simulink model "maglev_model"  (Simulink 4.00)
settings: Solver=ode45  StartTime=0.0  StopTime=10.0  RelTol=1e-3
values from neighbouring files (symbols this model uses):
  C = C * 1e-5    [maglev_init.m]
  g = 9.80665    [maglev_init.m]
  L1 = L1/10    [maglev_init.m]
  m = m/100    [maglev_init.m]
  R = input('Inserire le prime due cifre (esclusi zeri) del proprio numero di matricola:\n\n')    [maglev_init.m]
  x1_0 = 0.1    [maglev_init.m]
  x2_0 = 0    [maglev_init.m]
  x3_0 = 0.2    [maglev_init.m]

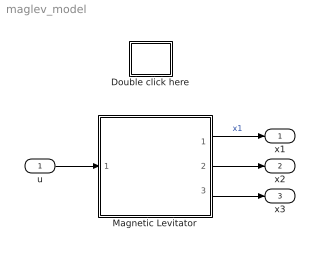
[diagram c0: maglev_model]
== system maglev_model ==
  u : Inport  Port=1  LatchInput=off
  Double click here : Subsystem
  Magnetic Levitator : Subsystem  mask{m=m, R=R, L1=L1, C=C, g=g}
      mask prompts: m "ball's mass (m)"; R "Electromagnet's resistance (R)"; L1 "Electromagnet's inductance (L1)"; C "Magnetic force constant (C)"; g "Gravitational acceleration (g)"
  x1 : Outport  Port=1
  x2 : Outport  Port=2
  x3 : Outport  Port=3
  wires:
  u/1 -> Magnetic Levitator/1(u)
  Magnetic Levitator/1(x1) -> x1/1  "x1"
  Magnetic Levitator/2(x2) -> x2/1
  Magnetic Levitator/3(x3) -> x3/1

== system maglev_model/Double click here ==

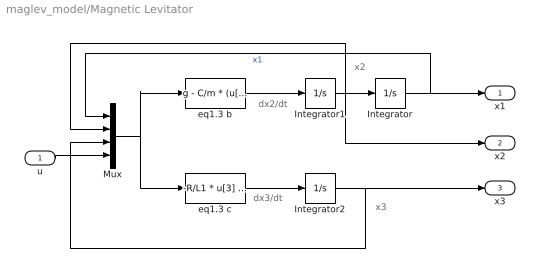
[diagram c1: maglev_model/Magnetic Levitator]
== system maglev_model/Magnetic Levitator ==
  note: x2
  note: x3
  note: dx2/dt
  note: dx3/dt
  u : Inport  Port=1  LatchInput=off
  Integrator : Integrator  ExternalReset=none  InitialConditionSource=internal  InitialCondition=x1_0  LimitOutput=off  UpperSaturationLimit=inf  LowerSaturationLimit=-inf  ShowSaturationPort=off  ShowStatePort=off  AbsoluteTolerance=auto
  Integrator1 : Integrator  ExternalReset=none  InitialConditionSource=internal  InitialCondition=x2_0  LimitOutput=off  UpperSaturationLimit=inf  LowerSaturationLimit=-inf  ShowSaturationPort=off  ShowStatePort=off  AbsoluteTolerance=auto
  Integrator2 : Integrator  ExternalReset=none  InitialConditionSource=internal  InitialCondition=x3_0  LimitOutput=off  UpperSaturationLimit=inf  LowerSaturationLimit=-inf  ShowSaturationPort=off  ShowStatePort=off  AbsoluteTolerance=auto
  Mux : Mux  Inputs=4
  eq1.3 b : Fcn  Expr=g - C/m * (u[3] / u[1])^2
  eq1.3 c : Fcn  Expr=-R/L1 * u[3] + (2*C)/L1 * ( u[2] * u[3] / u[1]^2 ) + 1/L1 * u[4]
  x1 : Outport  Port=1
  x2 : Outport  Port=2
  x3 : Outport  Port=3
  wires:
  eq1.3 b/1 -> Integrator1/1
  Integrator1/1 -> Integrator/1, Mux/2, x2/1
  eq1.3 c/1 -> Integrator2/1
  Mux/1 -> eq1.3 b/1, eq1.3 c/1
  Integrator/1 -> Mux/1, x1/1  "x1"
  Integrator2/1 -> Mux/3, x3/1
  u/1 -> Mux/4
